| stm32mp131_133_135 TFBGA320 11x11
[IBIS ver]   4.2
[File name]   stm32mp131_133_135_tfbga320.ibs
[File Rev]   3.4
[Date]   06-03-2024
[Source]   Data Created at STMicroelectronics
[Disclaimer]  This information is for modeling purpose only and is
   not guaranteed.
   The information is subject to change without notice.
[Copyright]   Copyright 2024 STMicroelectronics Inc.
|  You might uncomment [Merged Pins] sections if handeled by the simulation tool
[Component] stm32mp131_133_135_tfbga320
[Manufacturer] STMicroelectronics
[Package]
| variable   typ   min   max
R_pkg  0  NA  NA
L_pkg  0  NA  NA
C_pkg  0  NA  NA
[Pin]   signal_name   model_name
W17  BYPASS_REG1V8  nc
H20  DDR_A0  PDDRIO_PAD
N21  DDR_A1  PDDRIO_PAD
L18  DDR_A10  PDDRIO_PAD
N17  DDR_A11  PDDRIO_PAD
M19  DDR_A12  PDDRIO_PAD
G19  DDR_A13  PDDRIO_PAD
N19  DDR_A14  PDDRIO_PAD
M21  DDR_A15  PDDRIO_PAD
G20  DDR_A2  PDDRIO_PAD
H19  DDR_A3  PDDRIO_PAD
R19  DDR_A4  PDDRIO_PAD
F20  DDR_A5  PDDRIO_PAD
R21  DDR_A6  PDDRIO_PAD
J17  DDR_A7  PDDRIO_PAD
P19  DDR_A8  PDDRIO_PAD
G21  DDR_A9  PDDRIO_PAD
P18  DDR_ATO  nc
J19  DDR_BA0  PDDRIO_PAD
P20  DDR_BA1  PDDRIO_PAD
H18  DDR_BA2  PDDRIO_PAD
L19  DDR_CASN  PDDRIO_PAD
N20  DDR_CKE  PDDRIO_PAD
L20  DDR_CLKN  PDDRIO_PAD
M20  DDR_CLKP  PDDRIO_PAD
J20  DDR_CSN  PDDRIO_PAD
B21  DDR_DQ0  PDDRIO_PAD
B20  DDR_DQ1  PDDRIO_PAD
T19  DDR_DQ10  PDDRIO_PAD
W20  DDR_DQ11  PDDRIO_PAD
W19  DDR_DQ12  PDDRIO_PAD
U19  DDR_DQ13  PDDRIO_PAD
Y21  DDR_DQ14  PDDRIO_PAD
Y20  DDR_DQ15  PDDRIO_PAD
D19  DDR_DQ2  PDDRIO_PAD
E19  DDR_DQ3  PDDRIO_PAD
B19  DDR_DQ4  PDDRIO_PAD
D20  DDR_DQ5  PDDRIO_PAD
E20  DDR_DQ6  PDDRIO_PAD
F19  DDR_DQ7  PDDRIO_PAD
T20  DDR_DQ8  PDDRIO_PAD
U20  DDR_DQ9  PDDRIO_PAD
D21  DDR_DQM0  PDDRIO_PAD
W21  DDR_DQM1  PDDRIO_PAD
C21  DDR_DQS0N  PDIFF_PAD
C20  DDR_DQS0P  PDIFF_PAD
V21  DDR_DQS1N  PDIFF_PAD
V20  DDR_DQS1P  PDIFF_PAD
P17  DDR_DTO1  PDDRIO_PAD
J21  DDR_ODT  PDDRIO_PAD
K20  DDR_RASN  PDDRIO_PAD
H17  DDR_RESETN  PDDRIO_PAD
T18  DDR_VREF  nc
K19  DDR_WEN  PDDRIO_PAD
R20  DDR_ZQ  nc
V11  NJTRST  io8_ft
Y11  NRST  nc
W11  NRST_CORE  nc
Y3  PA0  io8_ft
AA3  PA1  io8_ft
AA19  PA10  io8usb_id_otg20_ft
Y1  PA11  io8_ft_i2c
F4  PA12  io8_ft_hslv
T4  PA13  io8_ft
W13  PA14  io8_ft
B4  PA15  io8_ft_hslv
Y4  PA2  io8_ft
W9  PA3  io8_ft_hslv
AA6  PA4  io8_ft
Y5  PA5  io8_ft
U10  PA6  io8_ft_hslv
V6  PA7  io8_ft_hslv
P2  PA8  io8_ft_i2c_hslv
A2  PA9  io8_ft_hslv
W8  PB0  io8_ft
Y8  PB1  io8_ft_hslv
E13  PB10  io8_ft_hslv
AA2  PB11  io8_ft_hslv_et
C11  PB12  io8_ft_hslv
D14  PB13  io8_ft_i2c_hslv
B16  PB14  io8_ft_hslv
B15  PB15  io8_ft_hslv
J3  PB2  io8_ft_hslv
C14  PB3  io8_ft_hslv
C16  PB4  io8_ft_hslv
B13  PB5  io8_ft_hslv
C1  PB6  io8_ft_hslv
C6  PB7  io8_ft_i2c
D1  PB8  io8_ft_i2c
A15  PB9  io8_ft_i2c_hslv
W5  PC0  io8_ft_hslv
Y9  PC1  io8_ft_hslv_et
A18  PC10  io8_ft_i2c_hslv
B18  PC11  io8_ft_i2c_hslv
A19  PC12  io8_ft_hslv
M3  PC13  io8_ft
M2  PC14  io8_ft
L3  PC15  io8_ft
AA10  PC2  io8_ft_hslv_et
W6  PC3  io8_ft_hslv
Y7  PC4  io8_ft
AA7  PC5  io8_ft
B14  PC6  io8_ft_hslv
C13  PC7  io8_ft_hslv
C18  PC8  io8_ft_hslv
A20  PC9  io8_ft_hslv
B1  PD0  io8_ft
C5  PD1  io8_ft_i2c_hslv
D6  PD10  io8_ft_hslv
F3  PD11  io8_ft_hslv
A6  PD12  io8_ft_i2c
J2  PD13  io8_ft_hslv
C4  PD14  io8_ft_i2c_hslv
E9  PD15  io8_ft_hslv
C19  PD2  io8_ft_hslv
C2  PD3  io8_ft_i2c
C7  PD4  io8_ft_hslv
C8  PD5  io8_ft_hslv
D2  PD6  io8_ft
V1  PD7  io8_ft_i2c_hslv
B5  PD8  io8_ft
C9  PD9  io8_ft_hslv
AA12  PDR_ON  nc
B6  PE0  io8_ft_hslv
E8  PE1  io8_ft_hslv
C10  PE10  io8_ft
B2  PE11  io8_ft_hslv_et
A4  PE12  io8_ft_hslv
A3  PE13  io8_ft_i2c_hslv
C3  PE14  io8_ft_hslv
A9  PE15  io8_ft_i2c_hslv
N1  PE2  io8_ft_i2c_hslv
B17  PE3  io8_ft_hslv
H2  PE4  io8_ft_hslv
W10  PE5  io8_ft_hslv_et
T2  PE6  io8_ft_hslv_et
D8  PE7  io8_ft_hslv
B9  PE8  io8_ft_i2c
B7  PE9  io8_ft_hslv
A16  PF0  io8_ft_hslv
B11  PF1  io8_ft_i2c_hslv
H3  PF10  io8_ft_hslv
Y6  PF11  io8_ft
AA4  PF12  io8_ft_hslv_et
W4  PF13  io8_ft
Y2  PF14  io8_ft
Y12  PF15  io8_ft
D11  PF2  io8_ft_i2c_hslv
A13  PF3  io8_ft_i2c_hslv
N2  PF4  io8_ft_hslv
B3  PF5  io8_ft_hslv
G1  PF6  io8_ft_hslv_et
P3  PF7  io8_ft_hslv_et
F1  PF8  io8_ft_hslv
J5  PF9  io8_ft_hslv
A7  PG0  io8_ft_hslv
R1  PG1  io8_ft_hslv_et
G2  PG10  io8_ft_hslv
R2  PG11  io8_ft_hslv_et
W2  PG12  io8_ft
AA9  PG13  io8_ft_hslv_et
Y10  PG14  io8_ft_hslv_et
H4  PG15  io8_ft_hslv
V3  PG2  io8_ft
W1  PG3  io8_ft_et_i2c_hslv
B10  PG4  io8_ft_hslv
G3  PG5  io8_ft_hslv
C17  PG6  io8_ft_hslv
A10  PG7  io8_ft_hslv
H5  PG8  io8_ft_hslv
F2  PG9  io8_ft_i2c
T3  PH0  io8_ft
U2  PH1  io8_ft
E14  PH10  io8_ft_hslv
K3  PH11  io8_ft_i2c_hslv
D3  PH12  io8_ft_i2c_hslv
A12  PH13  io8_ft_i2c_hslv
B8  PH14  io8_ft_i2c_hslv
E2  PH2  io8_ft_hslv
R3  PH3  io8_ft_i2c_hslv
Y19  PH4  io8_ft
W18  PH5  io8_ft
N3  PH6  io8_ft_i2c_hslv
J1  PH7  io8_ft_i2c_hslv
E3  PH8  io8_ft_i2c_hslv
C12  PH9  io8_ft_hslv
P5  PI0  io8_ft
P4  PI1  io8_ft
N5  PI2  io8_ft
L4  PI3  io8_ft
Y17  PI4  io8_ft
AA15  PI5  io8_ft
Y15  PI6  io8_ft
AA20  PI7  io8usb_vbus_otg20_ft
W3  PWR_CPU_ON  io8_ft
V19  PWR_LP  io8_ft
U17  PWR_ON  io8_ft
AA16  USB_DM1  nc
Y13  USB_DM2  nc
Y16  USB_DP1  nc
AA13  USB_DP2  nc
W12  USB_RREF  nc
L2  VBAT  power
V2  VDD_ANA  power
G11  VDD_CORE  power
J11  VDD_CORE  power
J15  VDD_CORE  power
L7  VDD_CORE  power
L9  VDD_CORE  power
L13  VDD_CORE  power
N10  VDD_CORE  power
N13  VDD_CORE  power
N15  VDD_CORE  power
R10  VDD_CORE  power
R13  VDD_CORE  power
U12  VDD_CORE  power
U14  VDD_CORE  power
E7  VDD_CPU  power
E10  VDD_CPU  power
G5  VDD_CPU  power
G7  VDD_CPU  power
G10  VDD_CPU  power
K5  VDD_CPU  power
K7  VDD_CPU  power
E15  VDD_DDR  power
G15  VDD_DDR  power
G17  VDD_DDR  power
K15  VDD_DDR  power
K17  VDD_DDR  power
M15  VDD_DDR  power
M17  VDD_DDR  power
R15  VDD_DDR  power
R17  VDD_DDR  power
U15  VDD_DDR  power
K2  VDD_PLL  power
Y18  VDD_PLL2  power
W14  VDD3V3_USBHS  power
U8  VDDA  power
V14  VDDA1V1_REG  power
W15  VDDA1V8_REG  power
E12  VDD  power
G9  VDD  power
G13  VDD  power
J7  VDD  power
J9  VDD  power
J13  VDD  power
E17  VDDSDMMC1  power
C15  VDDSDMMC2  power
M5  VDD  power
N7  VDD  power
N9  VDD  power
N12  VDD  power
R5  VDD  power
R7  VDD  power
R9  VDD  power
R12  VDD  power
U7  VDD  power
V8  VREFN  gnd
W7  VREFP  power
A1  VSS  gnd
A21  VSS  gnd
AA1  VSS  gnd
AA21  VSS  gnd
B12  VSS  gnd
D16  VSS  gnd
E5  VSS  gnd
E6  VSS  gnd
E11  VSS  gnd
E16  VSS  gnd
F5  VSS  gnd
F17  VSS  gnd
F18  VSS  gnd
F21  VSS  gnd
G8  VSS  gnd
G12  VSS  gnd
G14  VSS  gnd
H7  VSS  gnd
H15  VSS  gnd
J10  VSS  gnd
J12  VSS  gnd
K9  VSS  gnd
K10  VSS  gnd
K11  VSS  gnd
K12  VSS  gnd
K13  VSS  gnd
K21  VSS  gnd
L5  VSS  gnd
L10  VSS  gnd
L12  VSS  gnd
L15  VSS  gnd
L17  VSS  gnd
M1  VSS  gnd
M7  VSS  gnd
M9  VSS  gnd
M10  VSS  gnd
M11  VSS  gnd
M12  VSS  gnd
M13  VSS  gnd
N11  VSS  gnd
P7  VSS  gnd
P15  VSS  gnd
R8  VSS  gnd
R11  VSS  gnd
R14  VSS  gnd
T1  VSS  gnd
T5  VSS  gnd
T17  VSS  gnd
T21  VSS  gnd
U5  VSS  gnd
U6  VSS  gnd
U11  VSS  gnd
U16  VSS  gnd
V16  VSS  gnd
W16  VSS  gnd
U3  VSS_ANA  gnd
K1  VSS_PLL  gnd
AA18  VSS_PLL2  gnd
Y14  VSS_USBHS  gnd
U9  VSSA  gnd
U13  VSS  gnd
[Package Model]   501-bga-11x11-320-210615
[Pin Mapping]   pulldown_ref   pullup_ref   | Comment
W17  nc  nc  | Depending on IO usage
| W17  nc  nc  | Depending on IO usage
H20  gnd  vddddr
N21  gnd  vddddr
L18  gnd  vddddr
N17  gnd  vddddr
M19  gnd  vddddr
G19  gnd  vddddr
N19  gnd  vddddr
M21  gnd  vddddr
G20  gnd  vddddr
H19  gnd  vddddr
R19  gnd  vddddr
F20  gnd  vddddr
R21  gnd  vddddr
J17  gnd  vddddr
P19  gnd  vddddr
G21  gnd  vddddr
P18  nc  nc
J19  gnd  vddddr
P20  gnd  vddddr
H18  gnd  vddddr
L19  gnd  vddddr
N20  gnd  vddddr
L20  gnd  vddddr
M20  gnd  vddddr
J20  gnd  vddddr
B21  gnd  vddddr
B20  gnd  vddddr
T19  gnd  vddddr
W20  gnd  vddddr
W19  gnd  vddddr
U19  gnd  vddddr
Y21  gnd  vddddr
Y20  gnd  vddddr
D19  gnd  vddddr
E19  gnd  vddddr
B19  gnd  vddddr
D20  gnd  vddddr
E20  gnd  vddddr
F19  gnd  vddddr
T20  gnd  vddddr
U20  gnd  vddddr
D21  gnd  vddddr
W21  gnd  vddddr
C21  gnd  vddddr
C20  gnd  vddddr
V21  gnd  vddddr
V20  gnd  vddddr
P17  gnd  vddddr
J21  gnd  vddddr
K20  gnd  vddddr
H17  gnd  vddddr
T18  nc  nc
K19  gnd  vddddr
R20  nc  nc
V11  gnd  vddio
Y11  nc nc
W11  nc nc
Y3  gnd  vddio
AA3  gnd  vddio
AA19  gnd  vddio
Y1  gnd  vddio
F4  gnd  vddio
T4  gnd  vddio
W13  gnd  vddio
B4  gnd  vddio
Y4  gnd  vddio
W9  gnd  vddio
AA6  gnd  vddio
Y5  gnd  vddio
U10  gnd  vddio
V6  gnd  vddio
P2  gnd  vddio
A2  gnd  vddio
W8  gnd  vddio
Y8  gnd  vddio
E13  gnd  vddio
AA2  gnd  vddio
C11  gnd  vddio
D14  gnd  vddio
B16  gnd  vdds2  | Depending on IO usage
| B16  gnd  vddio  | Depending on IO usage
B15  gnd  vdds2  | Depending on IO usage
| B15  gnd  vddio  | Depending on IO usage
J3  gnd  vddio
C14  gnd  vdds2  | Depending on IO usage
| C14  gnd  vddio  | Depending on IO usage
C16  gnd  vdds2  | Depending on IO usage
| C16  gnd  vddio  | Depending on IO usage
B13  gnd  vddio
C1  gnd  vddio
C6  gnd  vddio
D1  gnd  vddio
A15  gnd  vddio
W5  gnd  vddio
Y9  gnd  vddio
A18  gnd  vdds1  | Depending on IO usage
| A18  gnd  vddio  | Depending on IO usage
B18  gnd  vdds1  | Depending on IO usage
| B18  gnd  vddio  | Depending on IO usage
A19  gnd  vdds1  | Depending on IO usage
| A19  gnd  vddio  | Depending on IO usage
M3  gnd  vddio  | Depending on IO usage
| M3  gnd  vbat  | Depending on IO usage
M2  gnd  vddio  | Depending on IO usage
| M2  gnd  vbat  | Depending on IO usage
L3  gnd  vddio  | Depending on IO usage
| L3  gnd  vbat  | Depending on IO usage
AA10  gnd  vddio
W6  gnd  vddio
Y7  gnd  vddio
AA7  gnd  vddio
B14  gnd  vddio
C13  gnd  vddio
C18  gnd  vdds1  | Depending on IO usage
| C18  gnd  vddio  | Depending on IO usage
A20  gnd  vdds1  | Depending on IO usage
| A20  gnd  vddio  | Depending on IO usage
B1  gnd  vddio
C5  gnd  vddio
D6  gnd  vddio
F3  gnd  vddio
A6  gnd  vddio
J2  gnd  vddio
C4  gnd  vddio
E9  gnd  vddio
C19  gnd  vdds1  | Depending on IO usage
| C19  gnd  vddio  | Depending on IO usage
C2  gnd  vddio
C7  gnd  vddio
C8  gnd  vddio
D2  gnd  vddio
V1  gnd  vddio
B5  gnd  vddio
C9  gnd  vddio
AA12  nc nc
B6  gnd  vddio
E8  gnd  vddio
C10  gnd  vddio
B2  gnd  vddio
A4  gnd  vddio
A3  gnd  vddio
C3  gnd  vddio
A9  gnd  vddio
N1  gnd  vddio
B17  gnd  vdds2  | Depending on IO usage
| B17  gnd  vddio  | Depending on IO usage
H2  gnd  vddio
W10  gnd  vddio
T2  gnd  vddio
D8  gnd  vddio
B9  gnd  vddio
B7  gnd  vddio
A16  gnd  vddio
B11  gnd  vddio
H3  gnd  vddio
Y6  gnd  vddio
AA4  gnd  vddio
W4  gnd  vddio
Y2  gnd  vddio
Y12  gnd  vddio
D11  gnd  vddio
A13  gnd  vddio
N2  gnd  vddio
B3  gnd  vddio
G1  gnd  vddio
P3  gnd  vddio
F1  gnd  vddio
J5  gnd  vddio
A7  gnd  vddio
R1  gnd  vddio
G2  gnd  vddio
R2  gnd  vddio
W2  gnd  vddio
AA9  gnd  vddio
Y10  gnd  vddio
H4  gnd  vddio
V3  gnd  vddio
W1  gnd  vddio
B10  gnd  vddio
G3  gnd  vddio
C17  gnd  vdds2  | Depending on IO usage
| C17  gnd  vddio  | Depending on IO usage
A10  gnd  vddio
H5  gnd  vddio
F2  gnd  vddio
T3  gnd  vddio
U2  gnd  vddio
E14  gnd  vddio
K3  gnd  vddio
D3  gnd  vddio
A12  gnd  vddio
B8  gnd  vddio
E2  gnd  vddio
R3  gnd  vddio
Y19  gnd  vddio
W18  gnd  vddio
N3  gnd  vddio
J1  gnd  vddio
E3  gnd  vddio
C12  gnd  vddio
P5  gnd  vddio
P4  gnd  vddio  | Depending on IO usage
| P4  gnd  vbat  | Depending on IO usage
N5  gnd  vddio  | Depending on IO usage
| N5  gnd  vbat  | Depending on IO usage
L4  gnd  vddio  | Depending on IO usage
| L4  gnd  vbat  | Depending on IO usage
Y17  gnd  vddio
AA15  gnd  vddio
Y15  gnd  vddio
AA20  gnd  vddio
W3  gnd  vddio
V19  gnd  vddio
U17  gnd  vddio
AA16  nc  nc  | Depending on IO usage
| AA16  nc  nc  | Depending on IO usage
Y13  nc  nc  | Depending on IO usage
| Y13  nc  nc  | Depending on IO usage
Y16  nc  nc  | Depending on IO usage
| Y16  nc  nc  | Depending on IO usage
AA13  nc  nc  | Depending on IO usage
| AA13  nc  nc  | Depending on IO usage
W12  nc  nc  | Depending on IO usage
| W12  nc  nc  | Depending on IO usage
L2  nc  vbat
V2  nc  vddana
G11  nc  vddio  | Depending on IO usage
| G11  nc  vbat  | Depending on IO usage
J11  nc  vddio  | Depending on IO usage
| J11  nc  vbat  | Depending on IO usage
J15  nc  vddio  | Depending on IO usage
| J15  nc  vbat  | Depending on IO usage
L7  nc  vddio  | Depending on IO usage
| L7  nc  vbat  | Depending on IO usage
L9  nc  vddio  | Depending on IO usage
| L9  nc  vbat  | Depending on IO usage
L13  nc  vddio  | Depending on IO usage
| L13  nc  vbat  | Depending on IO usage
N10  nc  vddio  | Depending on IO usage
| N10  nc  vbat  | Depending on IO usage
N13  nc  vddio  | Depending on IO usage
| N13  nc  vbat  | Depending on IO usage
N15  nc  vddio  | Depending on IO usage
| N15  nc  vbat  | Depending on IO usage
R10  nc  vddio  | Depending on IO usage
| R10  nc  vbat  | Depending on IO usage
R13  nc  vddio  | Depending on IO usage
| R13  nc  vbat  | Depending on IO usage
U12  nc  vddio  | Depending on IO usage
| U12  nc  vbat  | Depending on IO usage
U14  nc  vddio  | Depending on IO usage
| U14  nc  vbat  | Depending on IO usage
E7  nc  vddcpu
E10  nc  vddcpu
G5  nc  vddcpu
G7  nc  vddcpu
G10  nc  vddcpu
K5  nc  vddcpu
K7  nc  vddcpu
E15  nc  vddddr
G15  nc  vddddr
G17  nc  vddddr
K15  nc  vddddr
K17  nc  vddddr
M15  nc  vddddr
M17  nc  vddddr
R15  nc  vddddr
R17  nc  vddddr
U15  nc  vddddr
K2  nc  vddpll
Y18  nc  vddpll2
W14  nc  vdd3v3usbhs
U8  nc  vdda
V14  nc  vdda1v1
W15  nc  vdda1v8
E12  nc  vddio
G9  nc  vddio
G13  nc  vddio
J7  nc  vddio
J9  nc  vddio
J13  nc  vddio
E17  nc  vdds1
C15  nc  vdds2
M5  nc  vddio
N7  nc  vddio
N9  nc  vddio
N12  nc  vddio
R5  nc  vddio
R7  nc  vddio
R9  nc  vddio
R12  nc  vddio
U7  nc  vddio
V8  gnd  nc
W7  nc  vddio
A1  gnd  nc
A21  gnd  nc
AA1  gnd  nc
AA21  gnd  nc
B12  gnd  nc
D16  gnd  nc
E5  gnd  nc
E6  gnd  nc
E11  gnd  nc
E16  gnd  nc
F5  gnd  nc
F17  gnd  nc
F18  gnd  nc
F21  gnd  nc
G8  gnd  nc
G12  gnd  nc
G14  gnd  nc
H7  gnd  nc
H15  gnd  nc
J10  gnd  nc
J12  gnd  nc
K9  gnd  nc
K10  gnd  nc
K11  gnd  nc
K12  gnd  nc
K13  gnd  nc
K21  gnd  nc
L5  gnd  nc
L10  gnd  nc
L12  gnd  nc
L15  gnd  nc
L17  gnd  nc
M1  gnd  nc
M7  gnd  nc
M9  gnd  nc
M10  gnd  nc
M11  gnd  nc
M12  gnd  nc
M13  gnd  nc
N11  gnd  nc
P7  gnd  nc
P15  gnd  nc
R8  gnd  nc
R11  gnd  nc
R14  gnd  nc
T1  gnd  nc
T5  gnd  nc
T17  gnd  nc
T21  gnd  nc
U5  gnd  nc
U6  gnd  nc
U11  gnd  nc
U16  gnd  nc
V16  gnd  nc
W16  gnd  nc
U3  gnd  nc
K1  gnd  nc
AA18  gnd  nc
Y14  gnd  nc
U9  gnd  nc
U13  gnd  nc
[Diff_pin]   inv_pin   vdiff   tdelay_typ   tdelay_min   tdelay_max
   M20   L20   0.320V   0ns   NA   NA   |CK
   C20   C21   0.320V   0ns   NA   NA   |DQS0
   V20   V21   0.320V   0ns   NA   NA   |DQS1
[Model Selector] PDIFF_PAD
MSD_D3RF2_18   DDR2 MSD_D3R_PDIFF Z0=18-Ohm
MSD_D3RF2_40   DDR2 MSD_D3R_PDIFF Z0=40-Ohm
MSD_D3RF2_48   DDR2 MSD_D3R_PDIFF Z0=48-Ohm
MSD_D3RF2_ODT150   DDR2 MSD_D3R_PDIFF cell 150-Ohm ODT Receiver
MSD_D3RF2_ODT50   DDR2 MSD_D3R_PDIFF cell 50-Ohm ODT Receiver
MSD_D3RF2_ODT75   DDR2 MSD_D3R_PDIFF cell 75-Ohm ODT Receiver
MSD_D3RF2_ODTOFF   DDR2 MSD_D3R_PDIFF cell ODT off Receiver
MSD_D3RF3_34   DDR3 MSD_D3R_PDIFF cell  Z0=34-Ohm
MSD_D3RF3_40   DDR3 MSD_D3R_PDIFF cell  Z0=40-Ohm
MSD_D3RF3_48   DDR3 MSD_D3R_PDIFF cell  Z0=48-Ohm
MSD_D3RF3L_34   DDR3L MSD_D3R_PDIFF cell  Z0=34-Ohm
MSD_D3RF3L_40   DDR3L MSD_D3R_PDIFF cell  Z0=40-Ohm
MSD_D3RF3L_48   DDR3L MSD_D3R_PDIFF cell  Z0=48-Ohm
MSD_D3RF3L_ODT120   DDR3L MSD_D3R_PDIFF cell 120-Ohm ODT Receiver
MSD_D3RF3L_ODT40   DDR3L MSD_D3R_PDIFF cell 40-Ohm ODT Receiver
MSD_D3RF3L_ODT60   DDR3L MSD_D3R_PDIFF cell 60-Ohm ODT Receiver
MSD_D3RF3L_ODTOFF   DDR3L MSD_D3R_PDIFF cell ODT off Receiver
MSD_D3RF3_ODT120   DDR3 MSD_D3R_PDIFF cell 120-Ohm ODT Receiver
MSD_D3RF3_ODT40   DDR3 MSD_D3R_PDIFF cell 40-Ohm ODT Receiver
MSD_D3RF3_ODT60   DDR3 MSD_D3R_PDIFF cell 60-Ohm ODT Receiver
MSD_D3RF3_ODTOFF   DDR3 MSD_D3R_PDIFF cell ODT off Receiver
MSD_D3RFL2_34   LPDDR2 MSD_D3R_PDIFF cell  Z0=34-Ohm
MSD_D3RFL2_40   LPDDR2 MSD_D3R_PDIFF cell  Z0=40-Ohm
MSD_D3RFL2_48   LPDDR2 MSD_D3R_PDIFF cell  Z0=48-Ohm
MSD_D3RFL2_60   LPDDR2 MSD_D3R_PDIFF cell  Z0=60-Ohm
MSD_D3RFL2_80   LPDDR2 MSD_D3R_PDIFF cell  Z0=80-Ohm
MSD_D3RFL2_ODTOFF   LPDDR2 MSD_D3R_PDIFF cell ODT off Receiver
MSD_D3RFL_48   LPDDR MSD_D3R_PDIFF cell  Z0=48-Ohm
MSD_D3RFL_ODTOFF   LPDDR MSD_D3R_PDIFF cell ODT off Receiver
MSD_D3RF2_18_OPEN   DDR2 MSD_D3R_PDIFF_PDQSR Z0=18-Ohm
MSD_D3RF2_40_OPEN   DDR2 MSD_D3R_PDIFF_PDQSR Z0=40-Ohm
MSD_D3RF2_48_OPEN   DDR2 MSD_D3R_PDIFF_PDQSR Z0=48-Ohm
MSD_D3RF2_18_PD344   DDR2 MSD_D3R_PDIFF_PDQSR Z0=18-Ohm
MSD_D3RF2_40_PD344   DDR2 MSD_D3R_PDIFF_PDQSR Z0=40-Ohm
MSD_D3RF2_48_PD344   DDR2 MSD_D3R_PDIFF_PDQSR Z0=48-Ohm
MSD_D3RF2_18_PD393   DDR2 MSD_D3R_PDIFF_PDQSR Z0=18-Ohm
MSD_D3RF2_40_PD393   DDR2 MSD_D3R_PDIFF_PDQSR Z0=40-Ohm
MSD_D3RF2_48_PD393   DDR2 MSD_D3R_PDIFF_PDQSR Z0=48-Ohm
MSD_D3RF2_18_PD458   DDR2 MSD_D3R_PDIFF_PDQSR Z0=18-Ohm
MSD_D3RF2_40_PD458   DDR2 MSD_D3R_PDIFF_PDQSR Z0=40-Ohm
MSD_D3RF2_48_PD458   DDR2 MSD_D3R_PDIFF_PDQSR Z0=48-Ohm
MSD_D3RF2_18_PD500   DDR2 MSD_D3R_PDIFF_PDQSR Z0=18-Ohm
MSD_D3RF2_40_PD500   DDR2 MSD_D3R_PDIFF_PDQSR Z0=40-Ohm
MSD_D3RF2_48_PD500   DDR2 MSD_D3R_PDIFF_PDQSR Z0=48-Ohm
MSD_D3RF2_18_PD550   DDR2 MSD_D3R_PDIFF_PDQSR Z0=18-Ohm
MSD_D3RF2_40_PD550   DDR2 MSD_D3R_PDIFF_PDQSR Z0=40-Ohm
MSD_D3RF2_48_PD550   DDR2 MSD_D3R_PDIFF_PDQSR Z0=48-Ohm
MSD_D3RF2_18_PD611   DDR2 MSD_D3R_PDIFF_PDQSR Z0=18-Ohm
MSD_D3RF2_40_PD611   DDR2 MSD_D3R_PDIFF_PDQSR Z0=40-Ohm
MSD_D3RF2_48_PD611   DDR2 MSD_D3R_PDIFF_PDQSR Z0=48-Ohm
MSD_D3RF2_18_PD688   DDR2 MSD_D3R_PDIFF_PDQSR Z0=18-Ohm
MSD_D3RF2_40_PD688   DDR2 MSD_D3R_PDIFF_PDQSR Z0=40-Ohm
MSD_D3RF2_48_PD688   DDR2 MSD_D3R_PDIFF_PDQSR Z0=48-Ohm
MSD_D3RF2_18_PU344   DDR2 MSD_D3R_PDIFF_PDQSR Z0=18-Ohm
MSD_D3RF2_40_PU344   DDR2 MSD_D3R_PDIFF_PDQSR Z0=40-Ohm
MSD_D3RF2_48_PU344   DDR2 MSD_D3R_PDIFF_PDQSR Z0=48-Ohm
MSD_D3RF2_18_PU393   DDR2 MSD_D3R_PDIFF_PDQSR Z0=18-Ohm
MSD_D3RF2_40_PU393   DDR2 MSD_D3R_PDIFF_PDQSR Z0=40-Ohm
MSD_D3RF2_48_PU393   DDR2 MSD_D3R_PDIFF_PDQSR Z0=48-Ohm
MSD_D3RF2_18_PU458   DDR2 MSD_D3R_PDIFF_PDQSR Z0=18-Ohm
MSD_D3RF2_40_PU458   DDR2 MSD_D3R_PDIFF_PDQSR Z0=40-Ohm
MSD_D3RF2_48_PU458   DDR2 MSD_D3R_PDIFF_PDQSR Z0=48-Ohm
MSD_D3RF2_18_PU500   DDR2 MSD_D3R_PDIFF_PDQSR Z0=18-Ohm
MSD_D3RF2_40_PU500   DDR2 MSD_D3R_PDIFF_PDQSR Z0=40-Ohm
MSD_D3RF2_48_PU500   DDR2 MSD_D3R_PDIFF_PDQSR Z0=48-Ohm
MSD_D3RF2_18_PU550   DDR2 MSD_D3R_PDIFF_PDQSR Z0=18-Ohm
MSD_D3RF2_40_PU550   DDR2 MSD_D3R_PDIFF_PDQSR Z0=40-Ohm
MSD_D3RF2_48_PU550   DDR2 MSD_D3R_PDIFF_PDQSR Z0=48-Ohm
MSD_D3RF2_18_PU611   DDR2 MSD_D3R_PDIFF_PDQSR Z0=18-Ohm
MSD_D3RF2_40_PU611   DDR2 MSD_D3R_PDIFF_PDQSR Z0=40-Ohm
MSD_D3RF2_48_PU611   DDR2 MSD_D3R_PDIFF_PDQSR Z0=48-Ohm
MSD_D3RF2_18_PU688   DDR2 MSD_D3R_PDIFF_PDQSR Z0=18-Ohm
MSD_D3RF2_40_PU688   DDR2 MSD_D3R_PDIFF_PDQSR Z0=40-Ohm
MSD_D3RF2_48_PU688   DDR2 MSD_D3R_PDIFF_PDQSR Z0=48-Ohm
MSD_D3RF2_18_PWRDWN   DDR2 MSD_D3R_PDIFF_PDQSR Z0=18-Ohm
MSD_D3RF2_40_PWRDWN   DDR2 MSD_D3R_PDIFF_PDQSR Z0=40-Ohm
MSD_D3RF2_48_PWRDWN   DDR2 MSD_D3R_PDIFF_PDQSR Z0=48-Ohm
MSD_D3RF3_34_OPEN   DDR3 MSD_D3R_PDIFF_PDQSR cell  Z0=34-Ohm
MSD_D3RF3_40_OPEN   DDR3 MSD_D3R_PDIFF_PDQSR cell  Z0=40-Ohm
MSD_D3RF3_48_OPEN   DDR3 MSD_D3R_PDIFF_PDQSR cell  Z0=48-Ohm
MSD_D3RF3_34_PD344   DDR3 MSD_D3R_PDIFF_PDQSR cell  Z0=34-Ohm
MSD_D3RF3_40_PD344   DDR3 MSD_D3R_PDIFF_PDQSR cell  Z0=40-Ohm
MSD_D3RF3_48_PD344   DDR3 MSD_D3R_PDIFF_PDQSR cell  Z0=48-Ohm
MSD_D3RF3_34_PD393   DDR3 MSD_D3R_PDIFF_PDQSR cell  Z0=34-Ohm
MSD_D3RF3_40_PD393   DDR3 MSD_D3R_PDIFF_PDQSR cell  Z0=40-Ohm
MSD_D3RF3_48_PD393   DDR3 MSD_D3R_PDIFF_PDQSR cell  Z0=48-Ohm
MSD_D3RF3_34_PD458   DDR3 MSD_D3R_PDIFF_PDQSR cell  Z0=34-Ohm
MSD_D3RF3_40_PD458   DDR3 MSD_D3R_PDIFF_PDQSR cell  Z0=40-Ohm
MSD_D3RF3_48_PD458   DDR3 MSD_D3R_PDIFF_PDQSR cell  Z0=48-Ohm
MSD_D3RF3_34_PD500   DDR3 MSD_D3R_PDIFF_PDQSR cell  Z0=34-Ohm
MSD_D3RF3_40_PD500   DDR3 MSD_D3R_PDIFF_PDQSR cell  Z0=40-Ohm
MSD_D3RF3_48_PD500   DDR3 MSD_D3R_PDIFF_PDQSR cell  Z0=48-Ohm
MSD_D3RF3_34_PD550   DDR3 MSD_D3R_PDIFF_PDQSR cell  Z0=34-Ohm
MSD_D3RF3_40_PD550   DDR3 MSD_D3R_PDIFF_PDQSR cell  Z0=40-Ohm
MSD_D3RF3_48_PD550   DDR3 MSD_D3R_PDIFF_PDQSR cell  Z0=48-Ohm
MSD_D3RF3_34_PD611   DDR3 MSD_D3R_PDIFF_PDQSR cell  Z0=34-Ohm
MSD_D3RF3_40_PD611   DDR3 MSD_D3R_PDIFF_PDQSR cell  Z0=40-Ohm
MSD_D3RF3_48_PD611   DDR3 MSD_D3R_PDIFF_PDQSR cell  Z0=48-Ohm
MSD_D3RF3_34_PD688   DDR3 MSD_D3R_PDIFF_PDQSR cell  Z0=34-Ohm
MSD_D3RF3_40_PD688   DDR3 MSD_D3R_PDIFF_PDQSR cell  Z0=40-Ohm
MSD_D3RF3_48_PD688   DDR3 MSD_D3R_PDIFF_PDQSR cell  Z0=48-Ohm
MSD_D3RF3_34_PU344   DDR3 MSD_D3R_PDIFF_PDQSR cell  Z0=34-Ohm
MSD_D3RF3_40_PU344   DDR3 MSD_D3R_PDIFF_PDQSR cell  Z0=40-Ohm
MSD_D3RF3_48_PU344   DDR3 MSD_D3R_PDIFF_PDQSR cell  Z0=48-Ohm
MSD_D3RF3_34_PU393   DDR3 MSD_D3R_PDIFF_PDQSR cell  Z0=34-Ohm
MSD_D3RF3_40_PU393   DDR3 MSD_D3R_PDIFF_PDQSR cell  Z0=40-Ohm
MSD_D3RF3_48_PU393   DDR3 MSD_D3R_PDIFF_PDQSR cell  Z0=48-Ohm
MSD_D3RF3_34_PU458   DDR3 MSD_D3R_PDIFF_PDQSR cell  Z0=34-Ohm
MSD_D3RF3_40_PU458   DDR3 MSD_D3R_PDIFF_PDQSR cell  Z0=40-Ohm
MSD_D3RF3_48_PU458   DDR3 MSD_D3R_PDIFF_PDQSR cell  Z0=48-Ohm
MSD_D3RF3_34_PU500   DDR3 MSD_D3R_PDIFF_PDQSR cell  Z0=34-Ohm
MSD_D3RF3_40_PU500   DDR3 MSD_D3R_PDIFF_PDQSR cell  Z0=40-Ohm
MSD_D3RF3_48_PU500   DDR3 MSD_D3R_PDIFF_PDQSR cell  Z0=48-Ohm
MSD_D3RF3_34_PU550   DDR3 MSD_D3R_PDIFF_PDQSR cell  Z0=34-Ohm
MSD_D3RF3_40_PU550   DDR3 MSD_D3R_PDIFF_PDQSR cell  Z0=40-Ohm
MSD_D3RF3_48_PU550   DDR3 MSD_D3R_PDIFF_PDQSR cell  Z0=48-Ohm
MSD_D3RF3_34_PU611   DDR3 MSD_D3R_PDIFF_PDQSR cell  Z0=34-Ohm
MSD_D3RF3_40_PU611   DDR3 MSD_D3R_PDIFF_PDQSR cell  Z0=40-Ohm
MSD_D3RF3_48_PU611   DDR3 MSD_D3R_PDIFF_PDQSR cell  Z0=48-Ohm
MSD_D3RF3_34_PU688   DDR3 MSD_D3R_PDIFF_PDQSR cell  Z0=34-Ohm
MSD_D3RF3_40_PU688   DDR3 MSD_D3R_PDIFF_PDQSR cell  Z0=40-Ohm
MSD_D3RF3_48_PU688   DDR3 MSD_D3R_PDIFF_PDQSR cell  Z0=48-Ohm
MSD_D3RF3_34_PWRDWN   DDR3 MSD_D3R_PDIFF_PDQSR cell  Z0=34-Ohm
MSD_D3RF3_40_PWRDWN   DDR3 MSD_D3R_PDIFF_PDQSR cell  Z0=40-Ohm
MSD_D3RF3_48_PWRDWN   DDR3 MSD_D3R_PDIFF_PDQSR cell  Z0=48-Ohm
MSD_D3RF3L_34_OPEN   DDR3L MSD_D3R_PDIFF_PDQSR cell  Z0=34-Ohm
MSD_D3RF3L_40_OPEN   DDR3L MSD_D3R_PDIFF_PDQSR cell  Z0=40-Ohm
MSD_D3RF3L_48_OPEN   DDR3L MSD_D3R_PDIFF_PDQSR cell  Z0=48-Ohm
MSD_D3RF3L_34_PD344   DDR3L MSD_D3R_PDIFF_PDQSR cell  Z0=34-Ohm
MSD_D3RF3L_40_PD344   DDR3L MSD_D3R_PDIFF_PDQSR cell  Z0=40-Ohm
MSD_D3RF3L_48_PD344   DDR3L MSD_D3R_PDIFF_PDQSR cell  Z0=48-Ohm
MSD_D3RF3L_34_PD393   DDR3L MSD_D3R_PDIFF_PDQSR cell  Z0=34-Ohm
MSD_D3RF3L_40_PD393   DDR3L MSD_D3R_PDIFF_PDQSR cell  Z0=40-Ohm
MSD_D3RF3L_48_PD393   DDR3L MSD_D3R_PDIFF_PDQSR cell  Z0=48-Ohm
MSD_D3RF3L_34_PD458   DDR3L MSD_D3R_PDIFF_PDQSR cell  Z0=34-Ohm
MSD_D3RF3L_40_PD458   DDR3L MSD_D3R_PDIFF_PDQSR cell  Z0=40-Ohm
MSD_D3RF3L_48_PD458   DDR3L MSD_D3R_PDIFF_PDQSR cell  Z0=48-Ohm
MSD_D3RF3L_34_PD500   DDR3L MSD_D3R_PDIFF_PDQSR cell  Z0=34-Ohm
MSD_D3RF3L_40_PD500   DDR3L MSD_D3R_PDIFF_PDQSR cell  Z0=40-Ohm
MSD_D3RF3L_48_PD500   DDR3L MSD_D3R_PDIFF_PDQSR cell  Z0=48-Ohm
MSD_D3RF3L_34_PD550   DDR3L MSD_D3R_PDIFF_PDQSR cell  Z0=34-Ohm
MSD_D3RF3L_40_PD550   DDR3L MSD_D3R_PDIFF_PDQSR cell  Z0=40-Ohm
MSD_D3RF3L_48_PD550   DDR3L MSD_D3R_PDIFF_PDQSR cell  Z0=48-Ohm
MSD_D3RF3L_34_PD611   DDR3L MSD_D3R_PDIFF_PDQSR cell  Z0=34-Ohm
MSD_D3RF3L_40_PD611   DDR3L MSD_D3R_PDIFF_PDQSR cell  Z0=40-Ohm
MSD_D3RF3L_48_PD611   DDR3L MSD_D3R_PDIFF_PDQSR cell  Z0=48-Ohm
MSD_D3RF3L_34_PD688   DDR3L MSD_D3R_PDIFF_PDQSR cell  Z0=34-Ohm
MSD_D3RF3L_40_PD688   DDR3L MSD_D3R_PDIFF_PDQSR cell  Z0=40-Ohm
MSD_D3RF3L_48_PD688   DDR3L MSD_D3R_PDIFF_PDQSR cell  Z0=48-Ohm
MSD_D3RF3L_34_PU344   DDR3L MSD_D3R_PDIFF_PDQSR cell  Z0=34-Ohm
MSD_D3RF3L_40_PU344   DDR3L MSD_D3R_PDIFF_PDQSR cell  Z0=40-Ohm
MSD_D3RF3L_48_PU344   DDR3L MSD_D3R_PDIFF_PDQSR cell  Z0=48-Ohm
MSD_D3RF3L_34_PU393   DDR3L MSD_D3R_PDIFF_PDQSR cell  Z0=34-Ohm
MSD_D3RF3L_40_PU393   DDR3L MSD_D3R_PDIFF_PDQSR cell  Z0=40-Ohm
MSD_D3RF3L_48_PU393   DDR3L MSD_D3R_PDIFF_PDQSR cell  Z0=48-Ohm
MSD_D3RF3L_34_PU458   DDR3L MSD_D3R_PDIFF_PDQSR cell  Z0=34-Ohm
MSD_D3RF3L_40_PU458   DDR3L MSD_D3R_PDIFF_PDQSR cell  Z0=40-Ohm
MSD_D3RF3L_48_PU458   DDR3L MSD_D3R_PDIFF_PDQSR cell  Z0=48-Ohm
MSD_D3RF3L_34_PU500   DDR3L MSD_D3R_PDIFF_PDQSR cell  Z0=34-Ohm
MSD_D3RF3L_40_PU500   DDR3L MSD_D3R_PDIFF_PDQSR cell  Z0=40-Ohm
MSD_D3RF3L_48_PU500   DDR3L MSD_D3R_PDIFF_PDQSR cell  Z0=48-Ohm
MSD_D3RF3L_34_PU550   DDR3L MSD_D3R_PDIFF_PDQSR cell  Z0=34-Ohm
MSD_D3RF3L_40_PU550   DDR3L MSD_D3R_PDIFF_PDQSR cell  Z0=40-Ohm
MSD_D3RF3L_48_PU550   DDR3L MSD_D3R_PDIFF_PDQSR cell  Z0=48-Ohm
MSD_D3RF3L_34_PU611   DDR3L MSD_D3R_PDIFF_PDQSR cell  Z0=34-Ohm
MSD_D3RF3L_40_PU611   DDR3L MSD_D3R_PDIFF_PDQSR cell  Z0=40-Ohm
MSD_D3RF3L_48_PU611   DDR3L MSD_D3R_PDIFF_PDQSR cell  Z0=48-Ohm
MSD_D3RF3L_34_PU688   DDR3L MSD_D3R_PDIFF_PDQSR cell  Z0=34-Ohm
MSD_D3RF3L_40_PU688   DDR3L MSD_D3R_PDIFF_PDQSR cell  Z0=40-Ohm
MSD_D3RF3L_48_PU688   DDR3L MSD_D3R_PDIFF_PDQSR cell  Z0=48-Ohm
MSD_D3RF3L_34_PWRDWN   DDR3L MSD_D3R_PDIFF_PDQSR cell  Z0=34-Ohm
MSD_D3RF3L_40_PWRDWN   DDR3L MSD_D3R_PDIFF_PDQSR cell  Z0=40-Ohm
MSD_D3RF3L_48_PWRDWN   DDR3L MSD_D3R_PDIFF_PDQSR cell  Z0=48-Ohm
MSD_D3RFL2_34_OPEN   LPDDR2 MSD_D3R_PDIFF_PDQSR cell  Z0=34-Ohm
MSD_D3RFL2_40_OPEN   LPDDR2 MSD_D3R_PDIFF_PDQSR cell  Z0=40-Ohm
MSD_D3RFL2_48_OPEN   LPDDR2 MSD_D3R_PDIFF_PDQSR cell  Z0=48-Ohm
MSD_D3RFL2_60_OPEN   LPDDR2 MSD_D3R_PDIFF_PDQSR cell  Z0=60-Ohm
MSD_D3RFL2_80_OPEN   LPDDR2 MSD_D3R_PDIFF_PDQSR cell  Z0=80-Ohm
MSD_D3RFL_48_OPEN   LPDDR MSD_D3R_PDIFF_PDQSR cell  Z0=48-Ohm
MSD_D3RFL2_34_PD344   LPDDR2 MSD_D3R_PDIFF_PDQSR cell  Z0=34-Ohm
MSD_D3RFL2_40_PD344   LPDDR2 MSD_D3R_PDIFF_PDQSR cell  Z0=40-Ohm
MSD_D3RFL2_48_PD344   LPDDR2 MSD_D3R_PDIFF_PDQSR cell  Z0=48-Ohm
MSD_D3RFL2_60_PD344   LPDDR2 MSD_D3R_PDIFF_PDQSR cell  Z0=60-Ohm
MSD_D3RFL2_80_PD344   LPDDR2 MSD_D3R_PDIFF_PDQSR cell  Z0=80-Ohm
MSD_D3RFL_48_PD344   LPDDR MSD_D3R_PDIFF_PDQSR cell  Z0=48-Ohm
MSD_D3RFL2_34_PD393   LPDDR2 MSD_D3R_PDIFF_PDQSR cell  Z0=34-Ohm
MSD_D3RFL2_40_PD393   LPDDR2 MSD_D3R_PDIFF_PDQSR cell  Z0=40-Ohm
MSD_D3RFL2_48_PD393   LPDDR2 MSD_D3R_PDIFF_PDQSR cell  Z0=48-Ohm
MSD_D3RFL2_60_PD393   LPDDR2 MSD_D3R_PDIFF_PDQSR cell  Z0=60-Ohm
MSD_D3RFL2_80_PD393   LPDDR2 MSD_D3R_PDIFF_PDQSR cell  Z0=80-Ohm
MSD_D3RFL_48_PD393   LPDDR MSD_D3R_PDIFF_PDQSR cell  Z0=48-Ohm
MSD_D3RFL2_34_PD458   LPDDR2 MSD_D3R_PDIFF_PDQSR cell  Z0=34-Ohm
MSD_D3RFL2_40_PD458   LPDDR2 MSD_D3R_PDIFF_PDQSR cell  Z0=40-Ohm
MSD_D3RFL2_48_PD458   LPDDR2 MSD_D3R_PDIFF_PDQSR cell  Z0=48-Ohm
MSD_D3RFL2_60_PD458   LPDDR2 MSD_D3R_PDIFF_PDQSR cell  Z0=60-Ohm
MSD_D3RFL2_80_PD458   LPDDR2 MSD_D3R_PDIFF_PDQSR cell  Z0=80-Ohm
MSD_D3RFL_48_PD458   LPDDR MSD_D3R_PDIFF_PDQSR cell  Z0=48-Ohm
MSD_D3RFL2_34_PD500   LPDDR2 MSD_D3R_PDIFF_PDQSR cell  Z0=34-Ohm
MSD_D3RFL2_40_PD500   LPDDR2 MSD_D3R_PDIFF_PDQSR cell  Z0=40-Ohm
MSD_D3RFL2_48_PD500   LPDDR2 MSD_D3R_PDIFF_PDQSR cell  Z0=48-Ohm
MSD_D3RFL2_60_PD500   LPDDR2 MSD_D3R_PDIFF_PDQSR cell  Z0=60-Ohm
MSD_D3RFL2_80_PD500   LPDDR2 MSD_D3R_PDIFF_PDQSR cell  Z0=80-Ohm
MSD_D3RFL_48_PD500   LPDDR MSD_D3R_PDIFF_PDQSR cell  Z0=48-Ohm
MSD_D3RFL2_34_PD550   LPDDR2 MSD_D3R_PDIFF_PDQSR cell  Z0=34-Ohm
MSD_D3RFL2_40_PD550   LPDDR2 MSD_D3R_PDIFF_PDQSR cell  Z0=40-Ohm
MSD_D3RFL2_48_PD550   LPDDR2 MSD_D3R_PDIFF_PDQSR cell  Z0=48-Ohm
MSD_D3RFL2_60_PD550   LPDDR2 MSD_D3R_PDIFF_PDQSR cell  Z0=60-Ohm
MSD_D3RFL2_80_PD550   LPDDR2 MSD_D3R_PDIFF_PDQSR cell  Z0=80-Ohm
MSD_D3RFL_48_PD550   LPDDR MSD_D3R_PDIFF_PDQSR cell  Z0=48-Ohm
MSD_D3RFL2_34_PD611   LPDDR2 MSD_D3R_PDIFF_PDQSR cell  Z0=34-Ohm
MSD_D3RFL2_40_PD611   LPDDR2 MSD_D3R_PDIFF_PDQSR cell  Z0=40-Ohm
MSD_D3RFL2_48_PD611   LPDDR2 MSD_D3R_PDIFF_PDQSR cell  Z0=48-Ohm
MSD_D3RFL2_60_PD611   LPDDR2 MSD_D3R_PDIFF_PDQSR cell  Z0=60-Ohm
MSD_D3RFL2_80_PD611   LPDDR2 MSD_D3R_PDIFF_PDQSR cell  Z0=80-Ohm
MSD_D3RFL_48_PD611   LPDDR MSD_D3R_PDIFF_PDQSR cell  Z0=48-Ohm
MSD_D3RFL2_34_PD688   LPDDR2 MSD_D3R_PDIFF_PDQSR cell  Z0=34-Ohm
MSD_D3RFL2_40_PD688   LPDDR2 MSD_D3R_PDIFF_PDQSR cell  Z0=40-Ohm
MSD_D3RFL2_48_PD688   LPDDR2 MSD_D3R_PDIFF_PDQSR cell  Z0=48-Ohm
MSD_D3RFL2_60_PD688   LPDDR2 MSD_D3R_PDIFF_PDQSR cell  Z0=60-Ohm
MSD_D3RFL2_80_PD688   LPDDR2 MSD_D3R_PDIFF_PDQSR cell  Z0=80-Ohm
MSD_D3RFL_48_PD688   LPDDR MSD_D3R_PDIFF_PDQSR cell  Z0=48-Ohm
MSD_D3RFL2_34_PU344   LPDDR2 MSD_D3R_PDIFF_PDQSR cell  Z0=34-Ohm
MSD_D3RFL2_40_PU344   LPDDR2 MSD_D3R_PDIFF_PDQSR cell  Z0=40-Ohm
MSD_D3RFL2_48_PU344   LPDDR2 MSD_D3R_PDIFF_PDQSR cell  Z0=48-Ohm
MSD_D3RFL2_60_PU344   LPDDR2 MSD_D3R_PDIFF_PDQSR cell  Z0=60-Ohm
MSD_D3RFL2_80_PU344   LPDDR2 MSD_D3R_PDIFF_PDQSR cell  Z0=80-Ohm
MSD_D3RFL_48_PU344   LPDDR MSD_D3R_PDIFF_PDQSR cell  Z0=48-Ohm
MSD_D3RFL2_34_PU393   LPDDR2 MSD_D3R_PDIFF_PDQSR cell  Z0=34-Ohm
MSD_D3RFL2_40_PU393   LPDDR2 MSD_D3R_PDIFF_PDQSR cell  Z0=40-Ohm
MSD_D3RFL2_48_PU393   LPDDR2 MSD_D3R_PDIFF_PDQSR cell  Z0=48-Ohm
MSD_D3RFL2_60_PU393   LPDDR2 MSD_D3R_PDIFF_PDQSR cell  Z0=60-Ohm
MSD_D3RFL2_80_PU393   LPDDR2 MSD_D3R_PDIFF_PDQSR cell  Z0=80-Ohm
MSD_D3RFL_48_PU393   LPDDR MSD_D3R_PDIFF_PDQSR cell  Z0=48-Ohm
MSD_D3RFL2_34_PU458   LPDDR2 MSD_D3R_PDIFF_PDQSR cell  Z0=34-Ohm
MSD_D3RFL2_40_PU458   LPDDR2 MSD_D3R_PDIFF_PDQSR cell  Z0=40-Ohm
MSD_D3RFL2_48_PU458   LPDDR2 MSD_D3R_PDIFF_PDQSR cell  Z0=48-Ohm
MSD_D3RFL2_60_PU458   LPDDR2 MSD_D3R_PDIFF_PDQSR cell  Z0=60-Ohm
MSD_D3RFL2_80_PU458   LPDDR2 MSD_D3R_PDIFF_PDQSR cell  Z0=80-Ohm
MSD_D3RFL_48_PU458   LPDDR MSD_D3R_PDIFF_PDQSR cell  Z0=48-Ohm
MSD_D3RFL2_34_PU500   LPDDR2 MSD_D3R_PDIFF_PDQSR cell  Z0=34-Ohm
MSD_D3RFL2_40_PU500   LPDDR2 MSD_D3R_PDIFF_PDQSR cell  Z0=40-Ohm
MSD_D3RFL2_48_PU500   LPDDR2 MSD_D3R_PDIFF_PDQSR cell  Z0=48-Ohm
MSD_D3RFL2_60_PU500   LPDDR2 MSD_D3R_PDIFF_PDQSR cell  Z0=60-Ohm
MSD_D3RFL2_80_PU500   LPDDR2 MSD_D3R_PDIFF_PDQSR cell  Z0=80-Ohm
MSD_D3RFL_48_PU500   LPDDR MSD_D3R_PDIFF_PDQSR cell  Z0=48-Ohm
MSD_D3RFL2_34_PU550   LPDDR2 MSD_D3R_PDIFF_PDQSR cell  Z0=34-Ohm
MSD_D3RFL2_40_PU550   LPDDR2 MSD_D3R_PDIFF_PDQSR cell  Z0=40-Ohm
MSD_D3RFL2_48_PU550   LPDDR2 MSD_D3R_PDIFF_PDQSR cell  Z0=48-Ohm
MSD_D3RFL2_60_PU550   LPDDR2 MSD_D3R_PDIFF_PDQSR cell  Z0=60-Ohm
MSD_D3RFL2_80_PU550   LPDDR2 MSD_D3R_PDIFF_PDQSR cell  Z0=80-Ohm
MSD_D3RFL_48_PU550   LPDDR MSD_D3R_PDIFF_PDQSR cell  Z0=48-Ohm
MSD_D3RFL2_34_PU611   LPDDR2 MSD_D3R_PDIFF_PDQSR cell  Z0=34-Ohm
MSD_D3RFL2_40_PU611   LPDDR2 MSD_D3R_PDIFF_PDQSR cell  Z0=40-Ohm
MSD_D3RFL2_48_PU611   LPDDR2 MSD_D3R_PDIFF_PDQSR cell  Z0=48-Ohm
MSD_D3RFL2_60_PU611   LPDDR2 MSD_D3R_PDIFF_PDQSR cell  Z0=60-Ohm
MSD_D3RFL2_80_PU611   LPDDR2 MSD_D3R_PDIFF_PDQSR cell  Z0=80-Ohm
MSD_D3RFL_48_PU611   LPDDR MSD_D3R_PDIFF_PDQSR cell  Z0=48-Ohm
MSD_D3RFL2_34_PU688   LPDDR2 MSD_D3R_PDIFF_PDQSR cell  Z0=34-Ohm
MSD_D3RFL2_40_PU688   LPDDR2 MSD_D3R_PDIFF_PDQSR cell  Z0=40-Ohm
MSD_D3RFL2_48_PU688   LPDDR2 MSD_D3R_PDIFF_PDQSR cell  Z0=48-Ohm
MSD_D3RFL2_60_PU688   LPDDR2 MSD_D3R_PDIFF_PDQSR cell  Z0=60-Ohm
MSD_D3RFL2_80_PU688   LPDDR2 MSD_D3R_PDIFF_PDQSR cell  Z0=80-Ohm
MSD_D3RFL_48_PU688   LPDDR MSD_D3R_PDIFF_PDQSR cell  Z0=48-Ohm
MSD_D3RFL2_34_PWRDWN   LPDDR2 MSD_D3R_PDIFF_PDQSR cell  Z0=34-Ohm
MSD_D3RFL2_40_PWRDWN   LPDDR2 MSD_D3R_PDIFF_PDQSR cell  Z0=40-Ohm
MSD_D3RFL2_48_PWRDWN   LPDDR2 MSD_D3R_PDIFF_PDQSR cell  Z0=48-Ohm
MSD_D3RFL2_60_PWRDWN   LPDDR2 MSD_D3R_PDIFF_PDQSR cell  Z0=60-Ohm
MSD_D3RFL2_80_PWRDWN   LPDDR2 MSD_D3R_PDIFF_PDQSR cell  Z0=80-Ohm
MSD_D3RFL_48_PWRDWN   LPDDR MSD_D3R_PDIFF_PDQSR cell  Z0=48-Ohm
MSD_D3RF2_ODT150_OPEN   DDR2 MSD_D3R_PDIFF_PDQSR cell 150-Ohm ODT Receiver
MSD_D3RF2_ODT50_OPEN   DDR2 MSD_D3R_PDIFF_PDQSR cell 50-Ohm ODT Receiver
MSD_D3RF2_ODT75_OPEN   DDR2 MSD_D3R_PDIFF_PDQSR cell 75-Ohm ODT Receiver
MSD_D3RF2_ODTOFF_OPEN   DDR2 MSD_D3R_PDIFF_PDQSR cell ODT off Receiver
MSD_D3RF2_ODT150_PD344   DDR2 MSD_D3R_PDIFF_PDQSR cell 150-Ohm ODT Receiver
MSD_D3RF2_ODT50_PD344   DDR2 MSD_D3R_PDIFF_PDQSR cell 50-Ohm ODT Receiver
MSD_D3RF2_ODT75_PD344   DDR2 MSD_D3R_PDIFF_PDQSR cell 75-Ohm ODT Receiver
MSD_D3RF2_ODTOFF_PD344   DDR2 MSD_D3R_PDIFF_PDQSR cell ODT off Receiver
MSD_D3RF2_ODT150_PD393   DDR2 MSD_D3R_PDIFF_PDQSR cell 150-Ohm ODT Receiver
MSD_D3RF2_ODT50_PD393   DDR2 MSD_D3R_PDIFF_PDQSR cell 50-Ohm ODT Receiver
MSD_D3RF2_ODT75_PD393   DDR2 MSD_D3R_PDIFF_PDQSR cell 75-Ohm ODT Receiver
MSD_D3RF2_ODTOFF_PD393   DDR2 MSD_D3R_PDIFF_PDQSR cell ODT off Receiver
MSD_D3RF2_ODT150_PD458   DDR2 MSD_D3R_PDIFF_PDQSR cell 150-Ohm ODT Receiver
MSD_D3RF2_ODT50_PD458   DDR2 MSD_D3R_PDIFF_PDQSR cell 50-Ohm ODT Receiver
MSD_D3RF2_ODT75_PD458   DDR2 MSD_D3R_PDIFF_PDQSR cell 75-Ohm ODT Receiver
MSD_D3RF2_ODTOFF_PD458   DDR2 MSD_D3R_PDIFF_PDQSR cell ODT off Receiver
MSD_D3RF2_ODT150_PD500   DDR2 MSD_D3R_PDIFF_PDQSR cell 150-Ohm ODT Receiver
MSD_D3RF2_ODT50_PD500   DDR2 MSD_D3R_PDIFF_PDQSR cell 50-Ohm ODT Receiver
MSD_D3RF2_ODT75_PD500   DDR2 MSD_D3R_PDIFF_PDQSR cell 75-Ohm ODT Receiver
MSD_D3RF2_ODTOFF_PD500   DDR2 MSD_D3R_PDIFF_PDQSR cell ODT off Receiver
MSD_D3RF2_ODT150_PD550   DDR2 MSD_D3R_PDIFF_PDQSR cell 150-Ohm ODT Receiver
MSD_D3RF2_ODT50_PD550   DDR2 MSD_D3R_PDIFF_PDQSR cell 50-Ohm ODT Receiver
MSD_D3RF2_ODT75_PD550   DDR2 MSD_D3R_PDIFF_PDQSR cell 75-Ohm ODT Receiver
MSD_D3RF2_ODTOFF_PD550   DDR2 MSD_D3R_PDIFF_PDQSR cell ODT off Receiver
MSD_D3RF2_ODT150_PD611   DDR2 MSD_D3R_PDIFF_PDQSR cell 150-Ohm ODT Receiver
MSD_D3RF2_ODT50_PD611   DDR2 MSD_D3R_PDIFF_PDQSR cell 50-Ohm ODT Receiver
MSD_D3RF2_ODT75_PD611   DDR2 MSD_D3R_PDIFF_PDQSR cell 75-Ohm ODT Receiver
MSD_D3RF2_ODTOFF_PD611   DDR2 MSD_D3R_PDIFF_PDQSR cell ODT off Receiver
MSD_D3RF2_ODT150_PD688   DDR2 MSD_D3R_PDIFF_PDQSR cell 150-Ohm ODT Receiver
MSD_D3RF2_ODT50_PD688   DDR2 MSD_D3R_PDIFF_PDQSR cell 50-Ohm ODT Receiver
MSD_D3RF2_ODT75_PD688   DDR2 MSD_D3R_PDIFF_PDQSR cell 75-Ohm ODT Receiver
MSD_D3RF2_ODTOFF_PD688   DDR2 MSD_D3R_PDIFF_PDQSR cell ODT off Receiver
MSD_D3RF2_ODT150_PU344   DDR2 MSD_D3R_PDIFF_PDQSR cell 150-Ohm ODT Receiver
MSD_D3RF2_ODT50_PU344   DDR2 MSD_D3R_PDIFF_PDQSR cell 50-Ohm ODT Receiver
MSD_D3RF2_ODT75_PU344   DDR2 MSD_D3R_PDIFF_PDQSR cell 75-Ohm ODT Receiver
MSD_D3RF2_ODTOFF_PU344   DDR2 MSD_D3R_PDIFF_PDQSR cell ODT off Receiver
MSD_D3RF2_ODT150_PU393   DDR2 MSD_D3R_PDIFF_PDQSR cell 150-Ohm ODT Receiver
MSD_D3RF2_ODT50_PU393   DDR2 MSD_D3R_PDIFF_PDQSR cell 50-Ohm ODT Receiver
MSD_D3RF2_ODT75_PU393   DDR2 MSD_D3R_PDIFF_PDQSR cell 75-Ohm ODT Receiver
MSD_D3RF2_ODTOFF_PU393   DDR2 MSD_D3R_PDIFF_PDQSR cell ODT off Receiver
MSD_D3RF2_ODT150_PU458   DDR2 MSD_D3R_PDIFF_PDQSR cell 150-Ohm ODT Receiver
MSD_D3RF2_ODT50_PU458   DDR2 MSD_D3R_PDIFF_PDQSR cell 50-Ohm ODT Receiver
MSD_D3RF2_ODT75_PU458   DDR2 MSD_D3R_PDIFF_PDQSR cell 75-Ohm ODT Receiver
MSD_D3RF2_ODTOFF_PU458   DDR2 MSD_D3R_PDIFF_PDQSR cell ODT off Receiver
MSD_D3RF2_ODT150_PU500   DDR2 MSD_D3R_PDIFF_PDQSR cell 150-Ohm ODT Receiver
MSD_D3RF2_ODT50_PU500   DDR2 MSD_D3R_PDIFF_PDQSR cell 50-Ohm ODT Receiver
MSD_D3RF2_ODT75_PU500   DDR2 MSD_D3R_PDIFF_PDQSR cell 75-Ohm ODT Receiver
MSD_D3RF2_ODTOFF_PU500   DDR2 MSD_D3R_PDIFF_PDQSR cell ODT off Receiver
MSD_D3RF2_ODT150_PU550   DDR2 MSD_D3R_PDIFF_PDQSR cell 150-Ohm ODT Receiver
MSD_D3RF2_ODT50_PU550   DDR2 MSD_D3R_PDIFF_PDQSR cell 50-Ohm ODT Receiver
MSD_D3RF2_ODT75_PU550   DDR2 MSD_D3R_PDIFF_PDQSR cell 75-Ohm ODT Receiver
MSD_D3RF2_ODTOFF_PU550   DDR2 MSD_D3R_PDIFF_PDQSR cell ODT off Receiver
MSD_D3RF2_ODT150_PU611   DDR2 MSD_D3R_PDIFF_PDQSR cell 150-Ohm ODT Receiver
MSD_D3RF2_ODT50_PU611   DDR2 MSD_D3R_PDIFF_PDQSR cell 50-Ohm ODT Receiver
MSD_D3RF2_ODT75_PU611   DDR2 MSD_D3R_PDIFF_PDQSR cell 75-Ohm ODT Receiver
MSD_D3RF2_ODTOFF_PU611   DDR2 MSD_D3R_PDIFF_PDQSR cell ODT off Receiver
MSD_D3RF2_ODT150_PU688   DDR2 MSD_D3R_PDIFF_PDQSR cell 150-Ohm ODT Receiver
MSD_D3RF2_ODT50_PU688   DDR2 MSD_D3R_PDIFF_PDQSR cell 50-Ohm ODT Receiver
MSD_D3RF2_ODT75_PU688   DDR2 MSD_D3R_PDIFF_PDQSR cell 75-Ohm ODT Receiver
MSD_D3RF2_ODTOFF_PU688   DDR2 MSD_D3R_PDIFF_PDQSR cell ODT off Receiver
MSD_D3RF2_ODT150_PWRDWN   DDR2 MSD_D3R_PDIFF_PDQSR cell 150-Ohm ODT Receiver
MSD_D3RF2_ODT50_PWRDWN   DDR2 MSD_D3R_PDIFF_PDQSR cell 50-Ohm ODT Receiver
MSD_D3RF2_ODT75_PWRDWN   DDR2 MSD_D3R_PDIFF_PDQSR cell 75-Ohm ODT Receiver
MSD_D3RF2_ODTOFF_PWRDWN   DDR2 MSD_D3R_PDIFF_PDQSR cell ODT off Receiver
MSD_D3RF3_ODT120_OPEN   DDR3 MSD_D3R_PDIFF_PDQSR cell 120-Ohm ODT Receiver
MSD_D3RF3_ODT40_OPEN   DDR3 MSD_D3R_PDIFF_PDQSR cell 40-Ohm ODT Receiver
MSD_D3RF3_ODT60_OPEN   DDR3 MSD_D3R_PDIFF_PDQSR cell 60-Ohm ODT Receiver
MSD_D3RF3_ODTOFF_OPEN   DDR3 MSD_D3R_PDIFF_PDQSR cell ODT off Receiver
MSD_D3RF3_ODT120_PD344   DDR3 MSD_D3R_PDIFF_PDQSR cell 120-Ohm ODT Receiver
MSD_D3RF3_ODT40_PD344   DDR3 MSD_D3R_PDIFF_PDQSR cell 40-Ohm ODT Receiver
MSD_D3RF3_ODT60_PD344   DDR3 MSD_D3R_PDIFF_PDQSR cell 60-Ohm ODT Receiver
MSD_D3RF3_ODTOFF_PD344   DDR3 MSD_D3R_PDIFF_PDQSR cell ODT off Receiver
MSD_D3RF3_ODT120_PD393   DDR3 MSD_D3R_PDIFF_PDQSR cell 120-Ohm ODT Receiver
MSD_D3RF3_ODT40_PD393   DDR3 MSD_D3R_PDIFF_PDQSR cell 40-Ohm ODT Receiver
MSD_D3RF3_ODT60_PD393   DDR3 MSD_D3R_PDIFF_PDQSR cell 60-Ohm ODT Receiver
MSD_D3RF3_ODTOFF_PD393   DDR3 MSD_D3R_PDIFF_PDQSR cell ODT off Receiver
MSD_D3RF3_ODT120_PD458   DDR3 MSD_D3R_PDIFF_PDQSR cell 120-Ohm ODT Receiver
MSD_D3RF3_ODT40_PD458   DDR3 MSD_D3R_PDIFF_PDQSR cell 40-Ohm ODT Receiver
MSD_D3RF3_ODT60_PD458   DDR3 MSD_D3R_PDIFF_PDQSR cell 60-Ohm ODT Receiver
MSD_D3RF3_ODTOFF_PD458   DDR3 MSD_D3R_PDIFF_PDQSR cell ODT off Receiver
MSD_D3RF3_ODT120_PD500   DDR3 MSD_D3R_PDIFF_PDQSR cell 120-Ohm ODT Receiver
MSD_D3RF3_ODT40_PD500   DDR3 MSD_D3R_PDIFF_PDQSR cell 40-Ohm ODT Receiver
MSD_D3RF3_ODT60_PD500   DDR3 MSD_D3R_PDIFF_PDQSR cell 60-Ohm ODT Receiver
MSD_D3RF3_ODTOFF_PD500   DDR3 MSD_D3R_PDIFF_PDQSR cell ODT off Receiver
MSD_D3RF3_ODT120_PD550   DDR3 MSD_D3R_PDIFF_PDQSR cell 120-Ohm ODT Receiver
MSD_D3RF3_ODT40_PD550   DDR3 MSD_D3R_PDIFF_PDQSR cell 40-Ohm ODT Receiver
MSD_D3RF3_ODT60_PD550   DDR3 MSD_D3R_PDIFF_PDQSR cell 60-Ohm ODT Receiver
MSD_D3RF3_ODTOFF_PD550   DDR3 MSD_D3R_PDIFF_PDQSR cell ODT off Receiver
MSD_D3RF3_ODT120_PD611   DDR3 MSD_D3R_PDIFF_PDQSR cell 120-Ohm ODT Receiver
MSD_D3RF3_ODT40_PD611   DDR3 MSD_D3R_PDIFF_PDQSR cell 40-Ohm ODT Receiver
MSD_D3RF3_ODT60_PD611   DDR3 MSD_D3R_PDIFF_PDQSR cell 60-Ohm ODT Receiver
MSD_D3RF3_ODTOFF_PD611   DDR3 MSD_D3R_PDIFF_PDQSR cell ODT off Receiver
MSD_D3RF3_ODT120_PD688   DDR3 MSD_D3R_PDIFF_PDQSR cell 120-Ohm ODT Receiver
MSD_D3RF3_ODT40_PD688   DDR3 MSD_D3R_PDIFF_PDQSR cell 40-Ohm ODT Receiver
MSD_D3RF3_ODT60_PD688   DDR3 MSD_D3R_PDIFF_PDQSR cell 60-Ohm ODT Receiver
MSD_D3RF3_ODTOFF_PD688   DDR3 MSD_D3R_PDIFF_PDQSR cell ODT off Receiver
MSD_D3RF3_ODT120_PU344   DDR3 MSD_D3R_PDIFF_PDQSR cell 120-Ohm ODT Receiver
MSD_D3RF3_ODT40_PU344   DDR3 MSD_D3R_PDIFF_PDQSR cell 40-Ohm ODT Receiver
MSD_D3RF3_ODT60_PU344   DDR3 MSD_D3R_PDIFF_PDQSR cell 60-Ohm ODT Receiver
MSD_D3RF3_ODTOFF_PU344   DDR3 MSD_D3R_PDIFF_PDQSR cell ODT off Receiver
MSD_D3RF3_ODT120_PU393   DDR3 MSD_D3R_PDIFF_PDQSR cell 120-Ohm ODT Receiver
MSD_D3RF3_ODT40_PU393   DDR3 MSD_D3R_PDIFF_PDQSR cell 40-Ohm ODT Receiver
MSD_D3RF3_ODT60_PU393   DDR3 MSD_D3R_PDIFF_PDQSR cell 60-Ohm ODT Receiver
MSD_D3RF3_ODTOFF_PU393   DDR3 MSD_D3R_PDIFF_PDQSR cell ODT off Receiver
MSD_D3RF3_ODT120_PU458   DDR3 MSD_D3R_PDIFF_PDQSR cell 120-Ohm ODT Receiver
MSD_D3RF3_ODT40_PU458   DDR3 MSD_D3R_PDIFF_PDQSR cell 40-Ohm ODT Receiver
MSD_D3RF3_ODT60_PU458   DDR3 MSD_D3R_PDIFF_PDQSR cell 60-Ohm ODT Receiver
MSD_D3RF3_ODTOFF_PU458   DDR3 MSD_D3R_PDIFF_PDQSR cell ODT off Receiver
MSD_D3RF3_ODT120_PU500   DDR3 MSD_D3R_PDIFF_PDQSR cell 120-Ohm ODT Receiver
MSD_D3RF3_ODT40_PU500   DDR3 MSD_D3R_PDIFF_PDQSR cell 40-Ohm ODT Receiver
MSD_D3RF3_ODT60_PU500   DDR3 MSD_D3R_PDIFF_PDQSR cell 60-Ohm ODT Receiver
MSD_D3RF3_ODTOFF_PU500   DDR3 MSD_D3R_PDIFF_PDQSR cell ODT off Receiver
MSD_D3RF3_ODT120_PU550   DDR3 MSD_D3R_PDIFF_PDQSR cell 120-Ohm ODT Receiver
MSD_D3RF3_ODT40_PU550   DDR3 MSD_D3R_PDIFF_PDQSR cell 40-Ohm ODT Receiver
MSD_D3RF3_ODT60_PU550   DDR3 MSD_D3R_PDIFF_PDQSR cell 60-Ohm ODT Receiver
MSD_D3RF3_ODTOFF_PU550   DDR3 MSD_D3R_PDIFF_PDQSR cell ODT off Receiver
MSD_D3RF3_ODT120_PU611   DDR3 MSD_D3R_PDIFF_PDQSR cell 120-Ohm ODT Receiver
MSD_D3RF3_ODT40_PU611   DDR3 MSD_D3R_PDIFF_PDQSR cell 40-Ohm ODT Receiver
MSD_D3RF3_ODT60_PU611   DDR3 MSD_D3R_PDIFF_PDQSR cell 60-Ohm ODT Receiver
MSD_D3RF3_ODTOFF_PU611   DDR3 MSD_D3R_PDIFF_PDQSR cell ODT off Receiver
MSD_D3RF3_ODT120_PU688   DDR3 MSD_D3R_PDIFF_PDQSR cell 120-Ohm ODT Receiver
MSD_D3RF3_ODT40_PU688   DDR3 MSD_D3R_PDIFF_PDQSR cell 40-Ohm ODT Receiver
MSD_D3RF3_ODT60_PU688   DDR3 MSD_D3R_PDIFF_PDQSR cell 60-Ohm ODT Receiver
MSD_D3RF3_ODTOFF_PU688   DDR3 MSD_D3R_PDIFF_PDQSR cell ODT off Receiver
MSD_D3RF3_ODT120_PWRDWN   DDR3 MSD_D3R_PDIFF_PDQSR cell 120-Ohm ODT Receiver
MSD_D3RF3_ODT40_PWRDWN   DDR3 MSD_D3R_PDIFF_PDQSR cell 40-Ohm ODT Receiver
MSD_D3RF3_ODT60_PWRDWN   DDR3 MSD_D3R_PDIFF_PDQSR cell 60-Ohm ODT Receiver
MSD_D3RF3_ODTOFF_PWRDWN   DDR3 MSD_D3R_PDIFF_PDQSR cell ODT off Receiver
MSD_D3RF3L_ODT120_OPEN   DDR3L MSD_D3R_PDIFF_PDQSR cell 120-Ohm ODT Receiver
MSD_D3RF3L_ODT40_OPEN   DDR3L MSD_D3R_PDIFF_PDQSR cell 40-Ohm ODT Receiver
MSD_D3RF3L_ODT60_OPEN   DDR3L MSD_D3R_PDIFF_PDQSR cell 60-Ohm ODT Receiver
MSD_D3RF3L_ODTOFF_OPEN   DDR3L MSD_D3R_PDIFF_PDQSR cell ODT off Receiver
MSD_D3RF3L_ODT120_PD344   DDR3L MSD_D3R_PDIFF_PDQSR cell 120-Ohm ODT Receiver
MSD_D3RF3L_ODT40_PD344   DDR3L MSD_D3R_PDIFF_PDQSR cell 40-Ohm ODT Receiver
MSD_D3RF3L_ODT60_PD344   DDR3L MSD_D3R_PDIFF_PDQSR cell 60-Ohm ODT Receiver
MSD_D3RF3L_ODTOFF_PD344   DDR3L MSD_D3R_PDIFF_PDQSR cell ODT off Receiver
MSD_D3RF3L_ODT120_PD393   DDR3L MSD_D3R_PDIFF_PDQSR cell 120-Ohm ODT Receiver
MSD_D3RF3L_ODT40_PD393   DDR3L MSD_D3R_PDIFF_PDQSR cell 40-Ohm ODT Receiver
MSD_D3RF3L_ODT60_PD393   DDR3L MSD_D3R_PDIFF_PDQSR cell 60-Ohm ODT Receiver
MSD_D3RF3L_ODTOFF_PD393   DDR3L MSD_D3R_PDIFF_PDQSR cell ODT off Receiver
MSD_D3RF3L_ODT120_PD458   DDR3L MSD_D3R_PDIFF_PDQSR cell 120-Ohm ODT Receiver
MSD_D3RF3L_ODT40_PD458   DDR3L MSD_D3R_PDIFF_PDQSR cell 40-Ohm ODT Receiver
MSD_D3RF3L_ODT60_PD458   DDR3L MSD_D3R_PDIFF_PDQSR cell 60-Ohm ODT Receiver
MSD_D3RF3L_ODTOFF_PD458   DDR3L MSD_D3R_PDIFF_PDQSR cell ODT off Receiver
MSD_D3RF3L_ODT120_PD500   DDR3L MSD_D3R_PDIFF_PDQSR cell 120-Ohm ODT Receiver
MSD_D3RF3L_ODT40_PD500   DDR3L MSD_D3R_PDIFF_PDQSR cell 40-Ohm ODT Receiver
MSD_D3RF3L_ODT60_PD500   DDR3L MSD_D3R_PDIFF_PDQSR cell 60-Ohm ODT Receiver
MSD_D3RF3L_ODTOFF_PD500   DDR3L MSD_D3R_PDIFF_PDQSR cell ODT off Receiver
MSD_D3RF3L_ODT120_PD550   DDR3L MSD_D3R_PDIFF_PDQSR cell 120-Ohm ODT Receiver
MSD_D3RF3L_ODT40_PD550   DDR3L MSD_D3R_PDIFF_PDQSR cell 40-Ohm ODT Receiver
MSD_D3RF3L_ODT60_PD550   DDR3L MSD_D3R_PDIFF_PDQSR cell 60-Ohm ODT Receiver
MSD_D3RF3L_ODTOFF_PD550   DDR3L MSD_D3R_PDIFF_PDQSR cell ODT off Receiver
MSD_D3RF3L_ODT120_PD611   DDR3L MSD_D3R_PDIFF_PDQSR cell 120-Ohm ODT Receiver
MSD_D3RF3L_ODT40_PD611   DDR3L MSD_D3R_PDIFF_PDQSR cell 40-Ohm ODT Receiver
MSD_D3RF3L_ODT60_PD611   DDR3L MSD_D3R_PDIFF_PDQSR cell 60-Ohm ODT Receiver
MSD_D3RF3L_ODTOFF_PD611   DDR3L MSD_D3R_PDIFF_PDQSR cell ODT off Receiver
MSD_D3RF3L_ODT120_PD688   DDR3L MSD_D3R_PDIFF_PDQSR cell 120-Ohm ODT Receiver
MSD_D3RF3L_ODT40_PD688   DDR3L MSD_D3R_PDIFF_PDQSR cell 40-Ohm ODT Receiver
MSD_D3RF3L_ODT60_PD688   DDR3L MSD_D3R_PDIFF_PDQSR cell 60-Ohm ODT Receiver
MSD_D3RF3L_ODTOFF_PD688   DDR3L MSD_D3R_PDIFF_PDQSR cell ODT off Receiver
MSD_D3RF3L_ODT120_PU344   DDR3L MSD_D3R_PDIFF_PDQSR cell 120-Ohm ODT Receiver
MSD_D3RF3L_ODT40_PU344   DDR3L MSD_D3R_PDIFF_PDQSR cell 40-Ohm ODT Receiver
MSD_D3RF3L_ODT60_PU344   DDR3L MSD_D3R_PDIFF_PDQSR cell 60-Ohm ODT Receiver
MSD_D3RF3L_ODTOFF_PU344   DDR3L MSD_D3R_PDIFF_PDQSR cell ODT off Receiver
MSD_D3RF3L_ODT120_PU393   DDR3L MSD_D3R_PDIFF_PDQSR cell 120-Ohm ODT Receiver
MSD_D3RF3L_ODT40_PU393   DDR3L MSD_D3R_PDIFF_PDQSR cell 40-Ohm ODT Receiver
MSD_D3RF3L_ODT60_PU393   DDR3L MSD_D3R_PDIFF_PDQSR cell 60-Ohm ODT Receiver
MSD_D3RF3L_ODTOFF_PU393   DDR3L MSD_D3R_PDIFF_PDQSR cell ODT off Receiver
MSD_D3RF3L_ODT120_PU458   DDR3L MSD_D3R_PDIFF_PDQSR cell 120-Ohm ODT Receiver
MSD_D3RF3L_ODT40_PU458   DDR3L MSD_D3R_PDIFF_PDQSR cell 40-Ohm ODT Receiver
MSD_D3RF3L_ODT60_PU458   DDR3L MSD_D3R_PDIFF_PDQSR cell 60-Ohm ODT Receiver
MSD_D3RF3L_ODTOFF_PU458   DDR3L MSD_D3R_PDIFF_PDQSR cell ODT off Receiver
MSD_D3RF3L_ODT120_PU500   DDR3L MSD_D3R_PDIFF_PDQSR cell 120-Ohm ODT Receiver
MSD_D3RF3L_ODT40_PU500   DDR3L MSD_D3R_PDIFF_PDQSR cell 40-Ohm ODT Receiver
MSD_D3RF3L_ODT60_PU500   DDR3L MSD_D3R_PDIFF_PDQSR cell 60-Ohm ODT Receiver
MSD_D3RF3L_ODTOFF_PU500   DDR3L MSD_D3R_PDIFF_PDQSR cell ODT off Receiver
MSD_D3RF3L_ODT120_PU550   DDR3L MSD_D3R_PDIFF_PDQSR cell 120-Ohm ODT Receiver
MSD_D3RF3L_ODT40_PU550   DDR3L MSD_D3R_PDIFF_PDQSR cell 40-Ohm ODT Receiver
MSD_D3RF3L_ODT60_PU550   DDR3L MSD_D3R_PDIFF_PDQSR cell 60-Ohm ODT Receiver
MSD_D3RF3L_ODTOFF_PU550   DDR3L MSD_D3R_PDIFF_PDQSR cell ODT off Receiver
MSD_D3RF3L_ODT120_PU611   DDR3L MSD_D3R_PDIFF_PDQSR cell 120-Ohm ODT Receiver
MSD_D3RF3L_ODT40_PU611   DDR3L MSD_D3R_PDIFF_PDQSR cell 40-Ohm ODT Receiver
MSD_D3RF3L_ODT60_PU611   DDR3L MSD_D3R_PDIFF_PDQSR cell 60-Ohm ODT Receiver
MSD_D3RF3L_ODTOFF_PU611   DDR3L MSD_D3R_PDIFF_PDQSR cell ODT off Receiver
MSD_D3RF3L_ODT120_PU688   DDR3L MSD_D3R_PDIFF_PDQSR cell 120-Ohm ODT Receiver
MSD_D3RF3L_ODT40_PU688   DDR3L MSD_D3R_PDIFF_PDQSR cell 40-Ohm ODT Receiver
MSD_D3RF3L_ODT60_PU688   DDR3L MSD_D3R_PDIFF_PDQSR cell 60-Ohm ODT Receiver
MSD_D3RF3L_ODTOFF_PU688   DDR3L MSD_D3R_PDIFF_PDQSR cell ODT off Receiver
MSD_D3RF3L_ODT120_PWRDWN   DDR3L MSD_D3R_PDIFF_PDQSR cell 120-Ohm ODT Receiver
MSD_D3RF3L_ODT40_PWRDWN   DDR3L MSD_D3R_PDIFF_PDQSR cell 40-Ohm ODT Receiver
MSD_D3RF3L_ODT60_PWRDWN   DDR3L MSD_D3R_PDIFF_PDQSR cell 60-Ohm ODT Receiver
MSD_D3RF3L_ODTOFF_PWRDWN   DDR3L MSD_D3R_PDIFF_PDQSR cell ODT off Receiver
MSD_D3RFL2_ODTOFF_OPEN   LPDDR2 MSD_D3R_PDIFF_PDQSR cell ODT off Receiver
MSD_D3RFL_ODTOFF_OPEN   LPDDR MSD_D3R_PDIFF_PDQSR cell ODT off Receiver
MSD_D3RFL2_ODTOFF_PD344   LPDDR2 MSD_D3R_PDIFF_PDQSR cell ODT off Receiver
MSD_D3RFL_ODTOFF_PD344   LPDDR MSD_D3R_PDIFF_PDQSR cell ODT off Receiver
MSD_D3RFL2_ODTOFF_PD393   LPDDR2 MSD_D3R_PDIFF_PDQSR cell ODT off Receiver
MSD_D3RFL_ODTOFF_PD393   LPDDR MSD_D3R_PDIFF_PDQSR cell ODT off Receiver
MSD_D3RFL2_ODTOFF_PD458   LPDDR2 MSD_D3R_PDIFF_PDQSR cell ODT off Receiver
MSD_D3RFL_ODTOFF_PD458   LPDDR MSD_D3R_PDIFF_PDQSR cell ODT off Receiver
MSD_D3RFL2_ODTOFF_PD500   LPDDR2 MSD_D3R_PDIFF_PDQSR cell ODT off Receiver
MSD_D3RFL_ODTOFF_PD500   LPDDR MSD_D3R_PDIFF_PDQSR cell ODT off Receiver
MSD_D3RFL2_ODTOFF_PD550   LPDDR2 MSD_D3R_PDIFF_PDQSR cell ODT off Receiver
MSD_D3RFL_ODTOFF_PD550   LPDDR MSD_D3R_PDIFF_PDQSR cell ODT off Receiver
MSD_D3RFL2_ODTOFF_PD611   LPDDR2 MSD_D3R_PDIFF_PDQSR cell ODT off Receiver
MSD_D3RFL_ODTOFF_PD611   LPDDR MSD_D3R_PDIFF_PDQSR cell ODT off Receiver
MSD_D3RFL2_ODTOFF_PD688   LPDDR2 MSD_D3R_PDIFF_PDQSR cell ODT off Receiver
MSD_D3RFL_ODTOFF_PD688   LPDDR MSD_D3R_PDIFF_PDQSR cell ODT off Receiver
MSD_D3RFL2_ODTOFF_PU344   LPDDR2 MSD_D3R_PDIFF_PDQSR cell ODT off Receiver
MSD_D3RFL_ODTOFF_PU344   LPDDR MSD_D3R_PDIFF_PDQSR cell ODT off Receiver
MSD_D3RFL2_ODTOFF_PU393   LPDDR2 MSD_D3R_PDIFF_PDQSR cell ODT off Receiver
MSD_D3RFL_ODTOFF_PU393   LPDDR MSD_D3R_PDIFF_PDQSR cell ODT off Receiver
MSD_D3RFL2_ODTOFF_PU458   LPDDR2 MSD_D3R_PDIFF_PDQSR cell ODT off Receiver
MSD_D3RFL_ODTOFF_PU458   LPDDR MSD_D3R_PDIFF_PDQSR cell ODT off Receiver
MSD_D3RFL2_ODTOFF_PU500   LPDDR2 MSD_D3R_PDIFF_PDQSR cell ODT off Receiver
MSD_D3RFL_ODTOFF_PU500   LPDDR MSD_D3R_PDIFF_PDQSR cell ODT off Receiver
MSD_D3RFL2_ODTOFF_PU550   LPDDR2 MSD_D3R_PDIFF_PDQSR cell ODT off Receiver
MSD_D3RFL_ODTOFF_PU550   LPDDR MSD_D3R_PDIFF_PDQSR cell ODT off Receiver
MSD_D3RFL2_ODTOFF_PU611   LPDDR2 MSD_D3R_PDIFF_PDQSR cell ODT off Receiver
MSD_D3RFL_ODTOFF_PU611   LPDDR MSD_D3R_PDIFF_PDQSR cell ODT off Receiver
MSD_D3RFL2_ODTOFF_PU688   LPDDR2 MSD_D3R_PDIFF_PDQSR cell ODT off Receiver
MSD_D3RFL_ODTOFF_PU688   LPDDR MSD_D3R_PDIFF_PDQSR cell ODT off Receiver
MSD_D3RFL2_ODTOFF_PWRDWN   LPDDR2 MSD_D3R_PDIFF_PDQSR cell ODT off Receiver
MSD_D3RFL_ODTOFF_PWRDWN   LPDDR MSD_D3R_PDIFF_PDQSR cell ODT off Receiver
[Model Selector] PDDRIO_PAD
MSD_D3RP2_18   DDR2 MSD_D3R_PDDRIO Z0=18-Ohm
MSD_D3RP2_40   DDR2 MSD_D3R_PDDRIO Z0=40-Ohm
MSD_D3RP2_48   DDR2 MSD_D3R_PDDRIO Z0=48-Ohm
MSD_D3RP2_ODT150   DDR2 MSD_D3R_PDDRIO cell 150-Ohm ODT Receiver
MSD_D3RP2_ODT50   DDR2 MSD_D3R_PDDRIO cell 50-Ohm ODT Receiver
MSD_D3RP2_ODT75   DDR2 MSD_D3R_PDDRIO cell 75-Ohm ODT Receiver
MSD_D3RP2_ODTOFF   DDR2 MSD_D3R_PDDRIO cell ODT off Receiver
MSD_D3RP3_34   DDR3 MSD_D3R_PDDRIO cell  Z0=34-Ohm
MSD_D3RP3_40   DDR3 MSD_D3R_PDDRIO cell  Z0=40-Ohm
MSD_D3RP3_48   DDR3 MSD_D3R_PDDRIO cell  Z0=48-Ohm
MSD_D3RP3L_34   DDR3L MSD_D3R_PDDRIO cell  Z0=34-Ohm
MSD_D3RP3L_40   DDR3L MSD_D3R_PDDRIO cell  Z0=40-Ohm
MSD_D3RP3L_48   DDR3L MSD_D3R_PDDRIO cell  Z0=48-Ohm
MSD_D3RP3L_ODT120   DDR3L MSD_D3R_PDDRIO cell 120-Ohm ODT Receiver
MSD_D3RP3L_ODT40   DDR3L MSD_D3R_PDDRIO cell 40-Ohm ODT Receiver
MSD_D3RP3L_ODT60   DDR3L MSD_D3R_PDDRIO cell 60-Ohm ODT Receiver
MSD_D3RP3L_ODTOFF   DDR3L MSD_D3R_PDDRIO cell ODT off Receiver
MSD_D3RP3_ODT120   DDR3 MSD_D3R_PDDRIO cell 120-Ohm ODT Receiver
MSD_D3RP3_ODT40   DDR3 MSD_D3R_PDDRIO cell 40-Ohm ODT Receiver
MSD_D3RP3_ODT60   DDR3 MSD_D3R_PDDRIO cell 60-Ohm ODT Receiver
MSD_D3RP3_ODTOFF   DDR3 MSD_D3R_PDDRIO cell ODT off Receiver
MSD_D3RPL2_34   LPDDR2 MSD_D3R_PDDRIO cell  Z0=34-Ohm
MSD_D3RPL2_40   LPDDR2 MSD_D3R_PDDRIO cell  Z0=40-Ohm
MSD_D3RPL2_48   LPDDR2 MSD_D3R_PDDRIO cell  Z0=48-Ohm
MSD_D3RPL2_60   LPDDR2 MSD_D3R_PDDRIO cell  Z0=60-Ohm
MSD_D3RPL2_80   LPDDR2 MSD_D3R_PDDRIO cell  Z0=80-Ohm
MSD_D3RPL2_ODTOFF   LPDDR2 MSD_D3R_PDDRIO cell ODT off Receiver
MSD_D3RPL_48   LPDDR MSD_D3R_PDDRIO cell  Z0=48-Ohm
MSD_D3RPL_ODTOFF   LPDDR MSD_D3R_PDDRIO cell ODT off Receiver
[Model Selector] io8_ft
io8_ft_ls_1v2   "GPIO - 5V tolerant - 1.2V range - Low speed"
io8_ft_ms_1v2   "GPIO - 5V tolerant - 1.2V range - Med speed"
io8_ft_hs_1v2   "GPIO - 5V tolerant - 1.2V range - High speed"
io8_ft_fs_1v2   "GPIO - 5V tolerant - 1.2V range - Fast speed"
io8_ft_hs_1v8   "GPIO - 5V tolerant - 1.8V range - High speed -"
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| Models and submodels in the file (574): io8_ft_ls_1v2 (I/O), io8_ft_ms_1v2 (I/O), io8_ft_fs_1v2 (I/O), io8_ft_hs_1v2 (I/O), io8_ft_ls_1v8 (I/O), io8_ft_ms_1v8 (I/O), io8_ft_fs_1v8 (I/O), io8_ft_hs_1v8 (I/O), io8_ft_ls_3v3 (I/O), io8_ft_ms_3v3 (I/O), io8_ft_fs_3v3 (I/O), io8_ft_hs_3v3 (I/O), io8_ft_hslv_et_ls_1v2 (I/O), io8_ft_hslv_et_ms_1v2 (I/O), io8_ft_hslv_et_fs_1v2 (I/O), io8_ft_hslv_et_hs_1v2 (I/O), io8_ft_hslv_et_ls_1v8 (I/O), io8_ft_hslv_et_ms_1v8 (I/O), io8_ft_hslv_et_fs_1v8 (I/O), io8_ft_hslv_et_hs_1v8 (I/O), io8_ft_hslv_et_ls_2v5 (I/O), io8_ft_hslv_et_ms_2v5 (I/O), io8_ft_hslv_et_fs_2v5 (I/O), io8_ft_hslv_et_hs_2v5 (I/O), io8_ft_hslv_ls_1v2 (I/O), io8_ft_hslv_ms_1v2 (I/O), io8_ft_hslv_fs_1v2 (I/O), io8_ft_hslv_hs_1v2 (I/O), io8_ft_hslv_ls_1v8 (I/O), io8_ft_hslv_ms_1v8 (I/O), io8_ft_hslv_fs_1v8 (I/O), io8_ft_hslv_hs_1v8 (I/O), io8_ft_hslv_ls_2v5 (I/O), io8_ft_hslv_ms_2v5 (I/O), io8_ft_hslv_fs_2v5 (I/O), io8_ft_hslv_hs_2v5 (I/O), io8_ft_i2c_ls_1v2 (I/O_open_drain), io8_ft_i2c_ms_1v2 (I/O_open_drain), io8_ft_i2c_fs_1v2 (I/O_open_drain), io8_ft_i2c_hs_1v2 (I/O_open_drain), io8_ft_i2c_ls_1v8 (I/O_open_drain), io8_ft_i2c_ms_1v8 (I/O_open_drain), io8_ft_i2c_fs_1v8 (I/O_open_drain), io8_ft_i2c_hs_1v8 (I/O_open_drain), io8_ft_i2c_ls_3v3 (I/O_open_drain), io8_ft_i2c_ms_3v3 (I/O_open_drain), io8_ft_i2c_fs_3v3 (I/O_open_drain), io8_ft_i2c_hs_3v3 (I/O_open_drain), io8usb_adp_3v3 (I/O), io8usb_vbus_3v3 (I/O), io8usb_id_ft_nopup (Input), io8usb_id_ft_pup (Input), MSD_D3RF2_18 (I/O), MSD_D3RF2_40 (I/O), MSD_D3RF2_48 (I/O), MSD_D3RF2_ODT150 (Input), MSD_D3RF2_ODT50 (Input), MSD_D3RF2_ODT75 (Input), MSD_D3RF2_ODTOFF (Input), MSD_D3RF3_34 (I/O), MSD_D3RF3_40 (I/O), MSD_D3RF3_48 (I/O), MSD_D3RF3L_34 (I/O), MSD_D3RF3L_40 (I/O), MSD_D3RF3L_48 (I/O), MSD_D3RF3L_ODT120 (Input), MSD_D3RF3L_ODT40 (Input), MSD_D3RF3L_ODT60 (Input), MSD_D3RF3L_ODTOFF (Input), MSD_D3RF3_ODT120 (Input), MSD_D3RF3_ODT40 (Input), MSD_D3RF3_ODT60 (Input), MSD_D3RF3_ODTOFF (Input), MSD_D3RFL2_34 (I/O), MSD_D3RFL2_40 (I/O), MSD_D3RFL2_48 (I/O), MSD_D3RFL2_60 (I/O), MSD_D3RFL2_80 (I/O), MSD_D3RFL2_ODTOFF (Input), MSD_D3RFL_48 (I/O)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
